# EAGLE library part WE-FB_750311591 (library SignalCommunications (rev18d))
WE-FB Flyback Transformer suitable for LT3573/ LT3574/ LT3575/ LT3748 Characteristics easy design in solution less external components needed small board space low cost no optocoupler needed! long term reliability voltage control no aging same external parts for different output voltages easy design of custom power supply due to standard circuit and change of transformers and two components for feedback loop Isolation voltage up to 2.5 kV Applications Isolated power design Sensor interfaces Isolated telecom converters Power over Ethernet Details see: http://katalog.we-online.de/en/pbs/WE-FB_Linear? Updated 2015-04-03 2015 (C) Wurth Elektronik
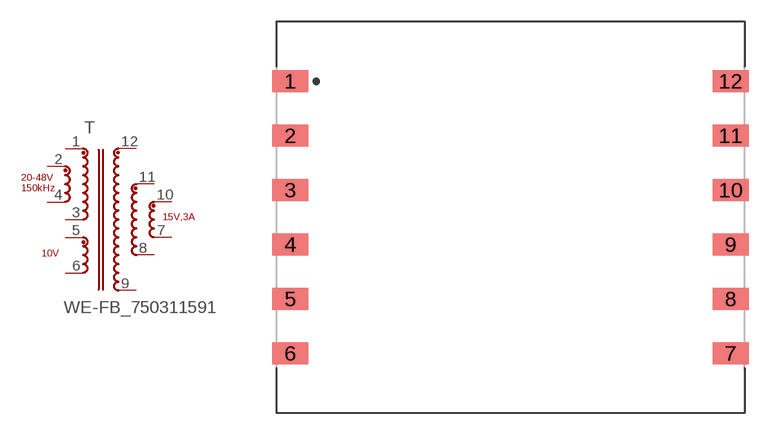
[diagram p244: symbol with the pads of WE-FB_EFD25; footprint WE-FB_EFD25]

Designator prefix T

## WE-FB_750311591  [WE-FB_EFD25]
1  2  pas
2  1  pas
3  11  pas
4  12  pas
5  10  pas
6  9  pas
7  6  pas
8  7  pas
9  8  pas
10  5  pas
11  4  pas
12  3  pas

## Footprint WE-FB_EFD25 (pad centres in mm)
smd 2.5 x 1.52: 1 -15.19,9.4; 2 -15.19,5.64; 3 -15.19,1.88; 4 -15.19,-1.88; 5 -15.19,-5.64; 6 -15.19,-9.4; 7 15.19,-9.4; 8 15.19,-5.64; 9 15.19,-1.88; 10 15.19,1.88; 11 15.19,5.64; 12 15.19,9.4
